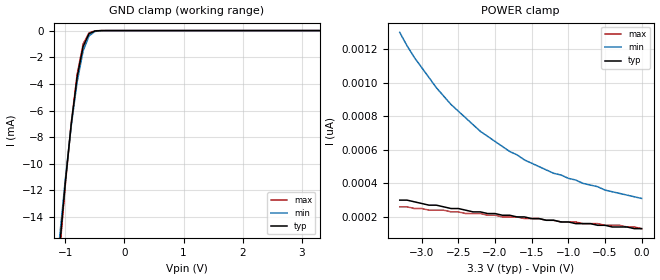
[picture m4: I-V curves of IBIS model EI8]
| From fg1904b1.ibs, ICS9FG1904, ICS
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|   Model EI8
[Model]   EI8
Model_type   Input
Polarity   Inverting
Vinl =   0.80V
Vinh =   2.00V
C_comp   3.40pF   2.85pF   3.95pF
[Temperature Range]   27.00   70.00   0.000
[Voltage Range]   3.30V   3.00V   3.70V
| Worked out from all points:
|   GND clamp passes 1 mA (typ) near -0.68 V on its own axis
[GND_clamp]
| voltage   I(typ)   I(min)   I(max)
-3.3V     -160mA     -150mA     -160mA
-1.1V     -16.38mA   -15.67mA   -16.85mA
-1V       -11.38mA   -11.14mA   -11.54mA
-900mV    -6.99mA    -7.13mA    -6.92mA
-800mV    -3.48mA    -3.84mA    -3.27mA
-700mV    -1.2mA     -1.54mA    -1.01mA
-600mV    -240uA     -400uA     -170uA
-500mV    -29.28uA   -66.42uA   -17.31uA
-400mV    -2.53uA    -8.31uA    -1.16uA
3.3V      160pA      130nA      110pA
[POWER_clamp]
| voltage   I(typ)   I(min)   I(max)
-3.3V     300pA      1.3nA      260pA
-3.1V     290pA      1.15nA     250pA
-2.9V     270pA      1.03nA     240pA
-2.8V     270pA      970pA      240pA
-2.6V     250pA      870pA      230pA
-2.2V     230pA      710pA      220pA
-1.8V     210pA      590pA      200pA
-1.2V     180pA      460pA      180pA
-900mV    160pA      420pA      170pA
-500mV    150pA      360pA      150pA
-300mV    140pA      340pA      150pA
0V        130pA      310pA      130pA
